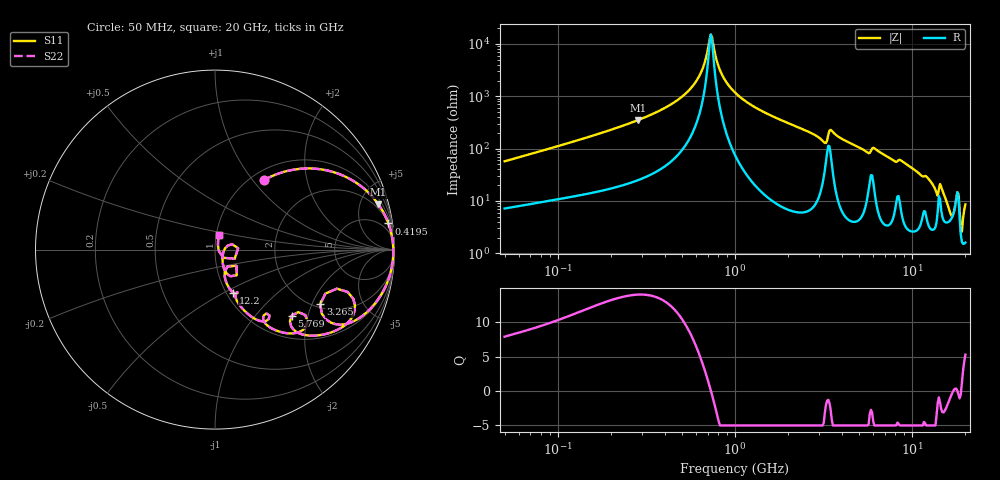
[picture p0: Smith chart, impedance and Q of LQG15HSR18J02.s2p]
!Murata Part Number: LQG15HSR18J02
!These Parameters are Measured in Series Mode Connection
!  o--[Z]--o
!Port1  Port2
!  o-------o
!Freq. Start=50[MHz] Stop=20[GHz], 401[Steps]
# Hz S RI R 50
!Freq.(Hz) S11(Real) S11(Imag) S21(Real) S21(Imag) S12(Real) S12(Imag) S22(Real) S22(Imag)
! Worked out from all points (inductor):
!   401 points, 50 MHz to 20 GHz, reference 50 ohm
!   read as one part in series: L = 178 nH near 51.52 MHz
!   highest Q = 14 at 284.2 MHz (marker M1), where L = 197 nH
!   self-resonance near 730.1 MHz
!   S11 on the Smith chart (normalised r, x): 50 MHz: 1.14, +1.14; 419.5 MHz: 2, +13; 3.265 GHz: 2.14, -2.31; 5.769 GHz: 1.48, -1.59; 12.2 GHz: 1.08, -0.56; 20 GHz: 1.03, +0.17
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5e7  0.2716 0.386  0.7284 -0.386  0.7284 -0.386  0.2716 0.386
1.364002e8  0.6851 0.4235  0.3149 -0.4235  0.3149 -0.4235  0.6851 0.4235
2.841629e8  0.9102 0.2524  0.0898 -0.2524  0.0898 -0.2524  0.9102 0.2524
3.721004e8  0.9527 0.1785  0.0473 -0.1785  0.0473 -0.1785  0.9527 0.1785
4.194704e8  0.966 0.146  0.034 -0.146  0.034 -0.146  0.966 0.146
6.009314e8  0.9895 0.0512  0.0105 -0.0512  0.0105 -0.0512  0.9895 0.0512
6.574395e8  0.9921 0.0278  0.00795 -0.0278  0.00795 -0.0278  0.9921 0.0278
7.30116e8  0.9935 0.000531  0.00652 -0.000531  0.00652 -0.000531  0.9935 0.000531
8.354841e8  0.9929 -0.0348  0.00711 0.0348  0.00711 0.0348  0.9929 -0.0348
1e9  0.9877 -0.083  0.0123 0.083  0.0123 0.083  0.9877 -0.083
2.728004e9  0.7821 -0.3945  0.2179 0.3945  0.2179 0.3945  0.7821 -0.3945
3.265178e9  0.5861 -0.3037  0.4139 0.3037  0.4139 0.3037  0.5861 -0.3037
3.626126e9  0.7698 -0.3649  0.2302 0.3649  0.2302 0.3649  0.7698 -0.3649
4.81993e9  0.5608 -0.4788  0.4392 0.4788  0.4392 0.4788  0.5608 -0.4788
5.769027e9  0.4281 -0.3675  0.5719 0.3675  0.5719 0.3675  0.4281 -0.3675
7.442007e9  0.3182 -0.4403  0.6818 0.4403  0.6818 0.4403  0.3182 -0.4403
1.220001e10  0.1028 -0.2401  0.8972 0.2401  0.8972 0.2401  0.1028 -0.2401
1.482269e10  0.0672 -0.1355  0.9328 0.1355  0.9328 0.1355  0.0672 -0.1355
1.670968e10  0.0449 -0.021  0.9551 0.021  0.9551 0.021  0.0449 -0.021
1.800918e10  0.1287 0.0078  0.8713 -0.0078  0.8713 -0.0078  0.1287 0.0078
1.912117e10  0.0166 0.0199  0.9834 -0.0199  0.9834 -0.0199  0.0166 0.0199
2e10  0.0226 0.0816  0.9774 -0.0816  0.9774 -0.0816  0.0226 0.0816
